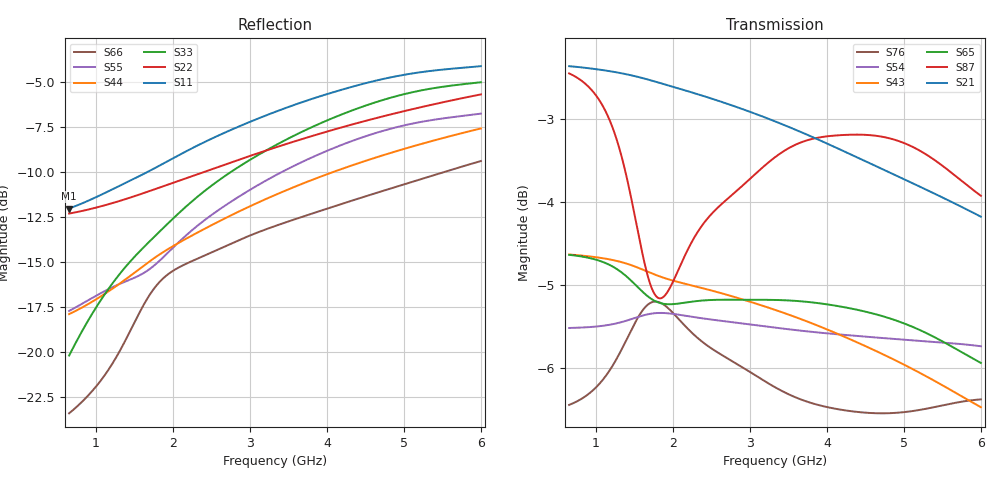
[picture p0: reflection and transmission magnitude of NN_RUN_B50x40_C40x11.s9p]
! IGNION VIRTUAL ANTENNA LIBRARY
! NN_RUN_B50x40_C40x11
! Virtual Antenna™ RUN mXTEND™: NN02-224 12.0 mm x 3.0 mm x 2.4 mm
! https://ignion.io/product/run-mxtend/
! Board: 50 mm x 40 mm
! Clearance Area: 40 mm x 11 mm
! Feeding line: L-shape; 11mm x 2mm and 5mm x 2mm
! Applications: Fleet management, IoT
! Frequency range 0.65GHz to 6GHz, step 10MHz
! Number of ports 9
! This product and its use is protected by at least one or more of the following patents and patent
! applications US 8,203,492 B2; US 8,237,615 B2; PCT/EP2013/064692; WO 2014/012842 A1; US 2019/190122 A1;
! US 62/072,671; and other domestic and international patents pending. Additional information about
! patents related to this product is available at https://ignion.io/files/Patent-list-NN.pdf, all
! rights reserved. Copyright, Ignion 2021.
! Need more help? Your platform is much different than these examples in the manual? Use our
! Fast Track service (https://ignion.io/fast-track/), for free, and get a personalized antenna design in
! just 24 hours.
! Touchstone port 1 = "Series Port"
! Touchstone port 2 = "Shunt Port"
! Touchstone port 3 = "Series Port"
! Touchstone port 4 = "Shunt Port"
! Touchstone port 5 = "Series Port"
! Touchstone port 6 = "Shunt Port"
! Touchstone port 7 = "Series Port"
! Touchstone port 8 = "Shunt Port"
! Touchstone port 9 = "Series Port"
! IE3D S-Parameters Output Version 2.0
# GHZ S MA R 50
! Nport = 9
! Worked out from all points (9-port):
!   536 points, 650 MHz to 6 GHz, reference 50 ohm
!   strongest paths, dB at 650 MHz, 1.99 GHz, 3.33 GHz, 4.67 GHz, 6 GHz:
!     S21: -2.4, -2.6, -3.0, -3.6, -4.2
!     S87: -2.4, -5.0, -3.5, -3.2, -3.9
!     S65: -4.6, -5.2, -5.2, -5.4, -5.9
!     S43: -4.6, -4.9, -5.3, -5.8, -6.5
!     S54: -5.5, -5.4, -5.5, -5.6, -5.7
!     S76: -6.5, -5.3, -6.2, -6.6, -6.4
!   lowest |S11| = -12.0 dB at 650 MHz (marker M1), VSWR 1.67, Z = 31.1 + j7.69 ohm
!   |S11| at or under -10 dB: start of sweep to 1.676 GHz
